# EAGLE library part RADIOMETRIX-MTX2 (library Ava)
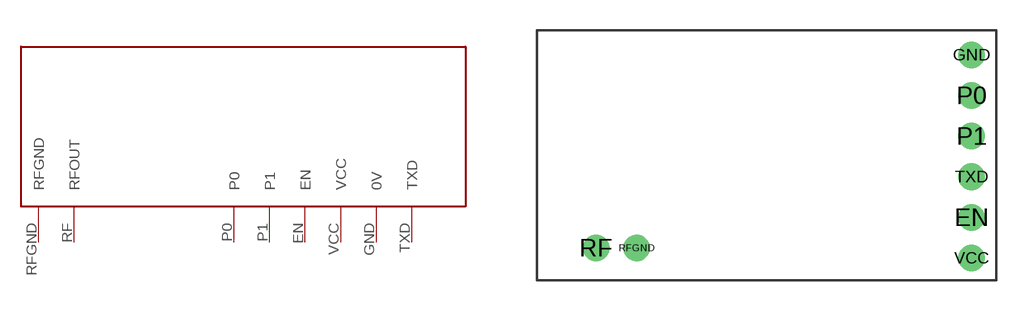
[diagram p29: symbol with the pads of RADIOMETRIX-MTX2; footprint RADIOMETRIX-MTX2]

Designator prefix -

## RADIOMETRIX-MTX2  [RADIOMETRIX-MTX2]
EN  EN
GND  0V
P0  P0
P1  P1
RF  RFOUT
RFGND  RFGND
TXD  TXD
VCC  VCC

## Footprint RADIOMETRIX-MTX2 (pad centres in mm)
drill 0.8: EN 9.97,-3.25; GND 9.97,4.75; P0 9.97,2.75; P1 9.97,0.75; RF -8.53,-4.75; RFGND -6.53,-4.75; TXD 9.97,-1.25; VCC 9.97,-5.25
